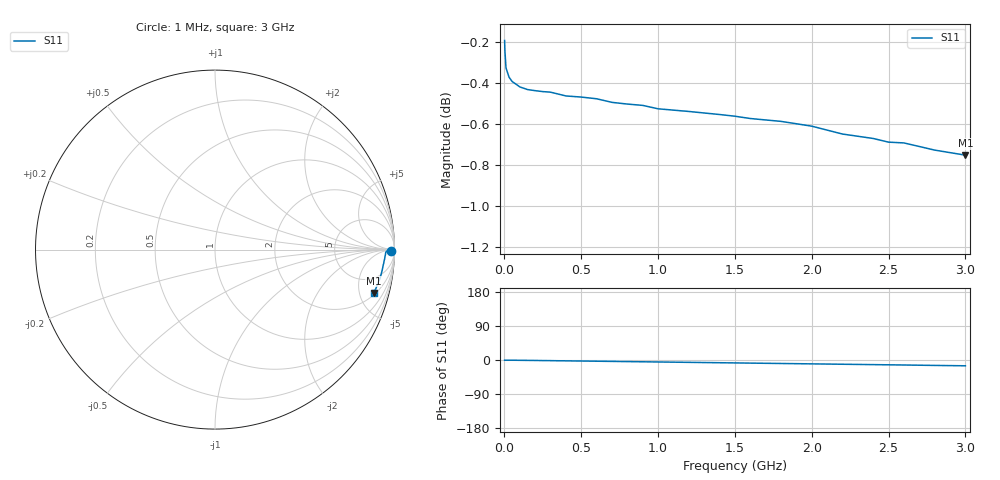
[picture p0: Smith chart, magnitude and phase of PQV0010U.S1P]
! SIEMENS Small Signal Semiconductors
! BAR64-04
! Si PIN Diode in SOT23 (2 diodes in series, pin 3 open)
! IF = 0.01 mA
! S-Parameters:  July  1992
# GHz  S  MA  R  50
!  f  S11
! GHz  MAG  ANG
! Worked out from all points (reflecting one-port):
!   33 points, 1 MHz to 3 GHz, reference 50 ohm
!   lowest |S11| = -0.8 dB at 3 GHz (marker M1), VSWR 23.13, Z = 111 - j337 ohm
!   phase of S11 starts at -0 deg and turns -15 deg over the sweep
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0.001  0.9779 -0.5
0.003  0.9723 -0.5
0.01  0.963 -0.5
0.03  0.958 -0.5
0.05  0.9557 -0.6
0.06  0.9551 -0.6
0.1  0.9528 -0.8
0.15  0.9514 -1.0
0.2  0.9508 -1.2
0.25  0.9503 -1.5
0.3  0.95 -1.7
0.35  0.949 -2.0
0.4  0.948 -2.2
0.45  0.9477 -2.5
0.5  0.9474 -2.7
0.8  0.9437 -4.2
0.9  0.943 -4.7
1  0.9412 -5.2
1.2  0.9398 -6.2
1.6  0.9361 -8.2
1.8  0.9346 -9.2
2  0.9321 -10.2
2.2  0.928 -11.2
2.4  0.9257 -12.2
2.5  0.9238 -12.7
2.6  0.9234 -13.2
2.8  0.9197 -14.3
3  0.9171 -15.3
